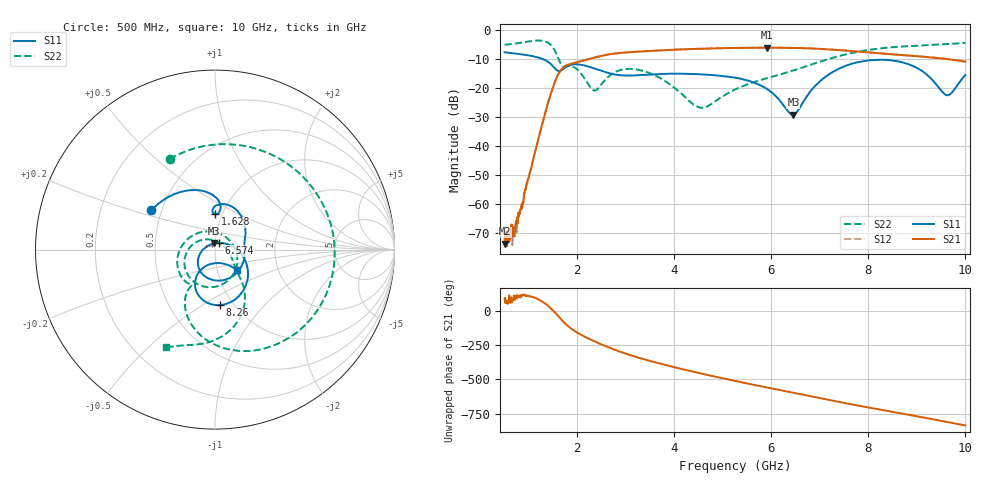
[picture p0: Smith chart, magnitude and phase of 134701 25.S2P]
!  2-Port S-parameters saved by WinCal
! VAR MeasName=S-Parameters (CALIBRATED_DATA) read from VNA (N5242A)
! VAR MeasDate=2013-7-3 16:32:26
! VAR NAME=134701 25
! VAR FILENAME=134701 25.S2P
! VAR DATE=2013-7-3 16:32:26
! VAR PHYS_PORTS=1,2
# Hz S MA R 50
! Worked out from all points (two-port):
!   1601 points, 500 MHz to 10 GHz, reference 50 ohm
!   highest |S21| = -6.00 dB at 5.915 GHz (marker M1); lowest = -73.8 dB at 511.9 MHz (marker M2)
!   |S21| within 3 dB of the highest: 2.452 GHz to 9.049 GHz (6.597 GHz wide, 115 % of centre)
!   lowest |S11| = -29.2 dB at 6.455 GHz (marker M3), VSWR 1.07, Z = 49.3 + j3.39 ohm
!   |S11| at or under -10 dB: 1.298 GHz to end of sweep
!   |S22| runs from -26.8 to -3.5 dB; largest |S21 - S12| = 0.0026
!   S11 on the Smith chart (normalised r, x): 500 MHz: 0.44, +0.23; 1.628 GHz: 0.93, +0.38; 6.574 GHz: 1.05, +0.08; 8.26 GHz: 0.87, -0.60; 10 GHz: 1.24, -0.30
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5e8  0.4176 148.3  0.0002546 80.9  0.0002341 61.1  0.5647 116.6
5.11875e8  0.4166 147.6  0.0002038 56.9  0.0001883 91.9  0.5655 114.9
7.078125e8  0.3987 136.0  0.0003957 92.9  0.0003965 101.8  0.5893 85.6
9.334375e8  0.376 122.0  0.00175 110.0  0.001759 111.0  0.6297 46.0
1.147188e9  0.3474 107.3  0.008922 91.0  0.009052 90.9  0.6667 0.2
1.396562e9  0.2859 88.0  0.05675 34.4  0.05672 34.3  0.6102 -65.8
1.628125e9  0.1976 89.3  0.188 -48.7  0.1878 -48.7  0.2985 -122.7
2.085312e9  0.2538 63.7  0.2948 -177.8  0.2947 -177.7  0.1747 166.8
2.358438e9  0.2184 41.4  0.3397 135.0  0.3401 135.1  0.09111 56.7
2.750312e9  0.174 18.1  0.3952 77.8  0.3953 77.7  0.1845 -65.6
3.670625e9  0.1754 -34.5  0.4492 -22.6  0.4489 -22.6  0.1552 -176.8
4.543438e9  0.1736 -84.7  0.4818 -97.0  0.4822 -97.1  0.04595 65.4
5.25e9  0.1519 -118.6  0.4958 -151.2  0.4964 -151.3  0.09484 -21.2
5.915e9  0.09601 -158.3  0.5013 160.4  0.501 160.3  0.1493 -41.8
6.455312e9  0.03476 99.1  0.4964 121.7  0.4972 121.6  0.203 -47.7
6.574062e9  0.04458 57.3  0.4937 113.3  0.4944 113.2  0.2186 -48.9
6.835312e9  0.09462 12.6  0.4862 94.7  0.4866 94.8  0.2581 -52.3
7.45875e9  0.23 -36.9  0.4523 51.5  0.4535 51.4  0.3716 -65.1
8.260312e9  0.3105 -84.6  0.3984 -0.9  0.3998 -1.2  0.489 -86.4
8.420625e9  0.3062 -93.1  0.3894 -11.2  0.3891 -11.4  0.5044 -90.3
9.614062e9  0.07544 -90.2  0.3203 -89.2  0.3191 -89.3  0.5779 -111.6
1e10  0.1691 -43.5  0.2886 -114.9  0.2876 -115.0  0.6082 -116.7
